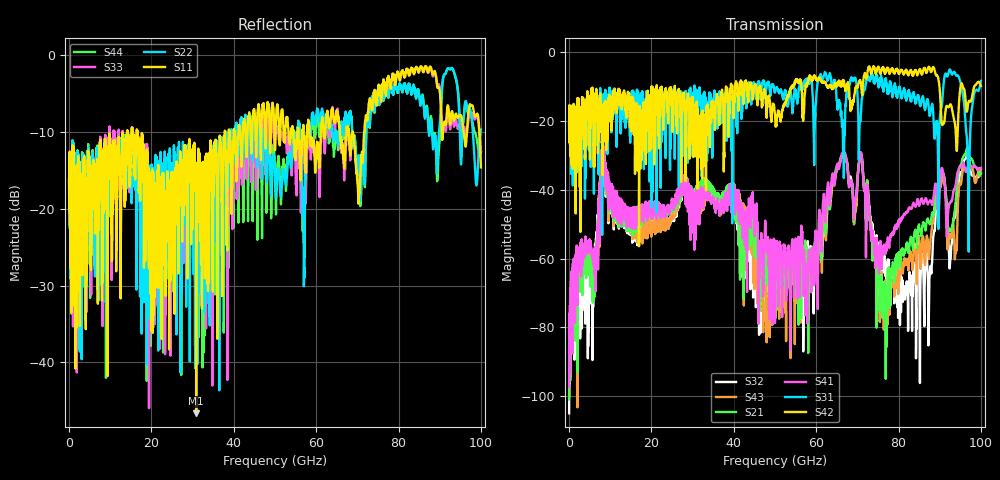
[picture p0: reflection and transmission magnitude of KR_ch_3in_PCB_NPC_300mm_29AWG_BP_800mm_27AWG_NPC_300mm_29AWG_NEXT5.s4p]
# GHz S RI R 45
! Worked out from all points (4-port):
!   4000 points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, 25 MHz to 100 GHz, reference 45 ohm
!   strongest paths, dB at 25 MHz, 25.02 GHz, 50.02 GHz, 75.03 GHz, 100 GHz:
!     S42: -20.6, -18.0, -18.0, -4.3, -9.8
!     S31: -20.7, -11.8, -11.4, -8.0, -8.3
!     S41: -97.4, -43.5, -74.9, -61.6, -33.6
!     S21: -101.0, -44.4, -63.5, -61.7, -35.0
!     S43: -99.8, -46.4, -70.4, -61.4, -34.1
!     S32: -105.0, -46.3, -72.2, -60.0, -35.3
!   lowest |S11| = -46.6 dB at 30.88 GHz (marker M1), VSWR 1.01, Z = 44.8 + j0.391 ohm
!   |S11| at or under -10 dB: start of sweep to 14.1 GHz; 16.57 GHz to 37.83 GHz (21.26 GHz wide, 78.2 % of centre); 68.94 GHz to 71.73 GHz (2.793 GHz wide, 3.97 % of centre)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
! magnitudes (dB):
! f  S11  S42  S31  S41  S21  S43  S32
! 25 MHz  -16.1  -20.6  -20.7  -97.4  -101.0  -99.8  -105.0
! 8.275 GHz  -14.5  -17.7  -16.4  -30.5  -31.3  -30.6  -31.4
! 30.88 GHz  -46.6  -30.3  -19.4  -39.8  -38.8  -42.7  -40.7
! 55.05 GHz  -13.7  -7.9  -10.9  -54.6  -59.9  -71.7  -61.9
! 70.8 GHz  -15.2  -8.5  -18.5  -29.1  -29.8  -29.0  -29.7
! 76.6 GHz  -3.4  -5.9  -9.8  -58.2  -70.9  -69.0  -61.2
! 100 GHz  -14.6  -9.8  -8.3  -33.6  -35.0  -34.1  -35.3
